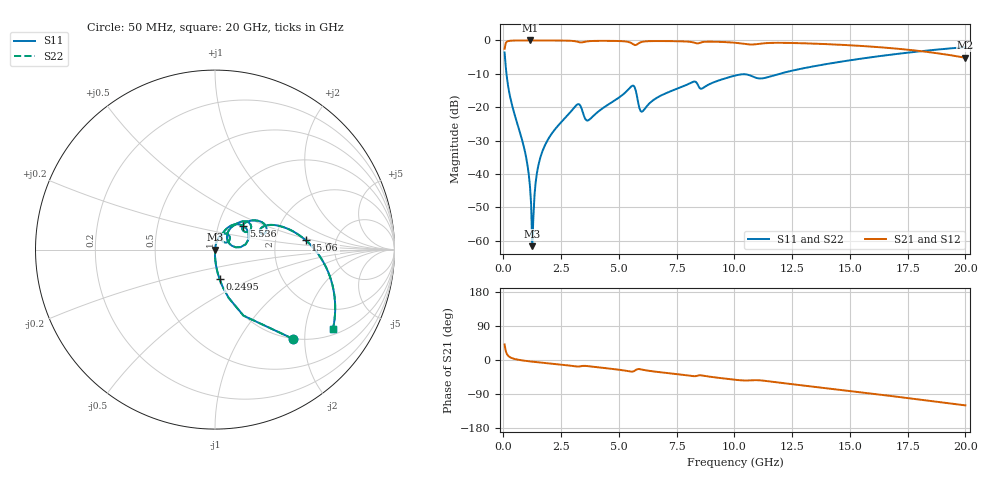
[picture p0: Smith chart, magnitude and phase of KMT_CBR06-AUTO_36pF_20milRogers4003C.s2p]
! Data measured by Modelithics Inc. support@modelithics.com 813-866-6335
! KEMET CBR06-AUTO 36pF, Pad Width= 0.851mm, Pad Length= 0.64mm, Pad Gap= 0.62mm, 20mil Rogers 4003C substrate Data, January 2022
# hz S ma R 50
! 2 Port Network Data from SP1.SP block
! freq  magS11  angS11  magS21  angS21  magS12  angS12  magS22  angS22
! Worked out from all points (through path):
!   401 points, 50 MHz to 20 GHz, reference 50 ohm
!   highest |S21| = -0.01 dB at 1.147 GHz (marker M1); lowest = -5.2 dB at 20 GHz (marker M2)
!   group delay of S21, straight-line fit = 16.7 ps
!   lowest |S11| = -61.6 dB at 1.247 GHz (marker M3), VSWR 1.00, Z = 50.1 - j0.0651 ohm
!   |S11| at or under -10 dB: 132.2 MHz to 11.95 GHz (11.82 GHz wide, 196 % of centre)
!   |S22| runs from -61.6 to -2.0 dB; largest |S21 - S12| = 0
!   S11 on the Smith chart (normalised r, x): 50 MHz: 1.00, -1.75; 249.5 MHz: 1.00, -0.34; 5.536 GHz: 1.32, +0.36; 15.06 GHz: 3.00, +0.42; 20 GHz: 1.17, -2.82
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5e7  0.6596 -48.9  0.7513 41.1  0.7513 41.1  0.6596 -48.9
2.495e8  0.167 -81.2  0.9856 8.7  0.9856 8.7  0.167 -81.2
9.4775e8  0.0203 -90.8  0.9993 -2.2  0.9993 -2.2  0.0203 -90.8
1.097375e9  0.009743 -90.3  0.9994 -3.3  0.9994 -3.3  0.009743 -90.3
1.14725e9  0.006579 -89.0  0.9994 -3.7  0.9994 -3.7  0.006579 -89.0
1.247e9  0.0008281 -51.7  0.9994 -4.4  0.9994 -4.4  0.0008281 -51.7
1.34675e9  0.004958 78.1  0.9993 -5.1  0.9993 -5.1  0.004958 78.1
1.4465e9  0.01015 80.8  0.9993 -5.7  0.9993 -5.7  0.01015 80.8
1.54625e9  0.01512 81.2  0.9992 -6.3  0.9992 -6.3  0.01512 81.2
1.8455e9  0.02912 80.2  0.9987 -8.2  0.9987 -8.2  0.02912 80.2
3.14225e9  0.1059 58.3  0.9678 -17.0  0.9678 -17.0  0.1059 58.3
3.391625e9  0.09361 32.0  0.9347 -16.0  0.9347 -16.0  0.09361 32.0
3.690875e9  0.06407 51.3  0.9738 -16.4  0.9738 -16.4  0.06407 51.3
5.53625e9  0.205 40.1  0.9134 -30.7  0.9134 -30.7  0.205 40.1
5.985125e9  0.0854 30.4  0.9489 -25.1  0.9489 -25.1  0.0854 30.4
6.73325e9  0.1441 54.1  0.9793 -31.9  0.9793 -31.9  0.1441 54.1
1.0025e10  0.2974 31.7  0.9233 -52.2  0.9233 -52.2  0.2974 31.7
1.1222e10  0.2707 22.6  0.9026 -54.3  0.9026 -54.3  0.2707 22.6
1.336662e10  0.4058 17.7  0.8977 -70.0  0.8977 -70.0  0.4058 17.7
1.506238e10  0.5078 5.9  0.8442 -82.2  0.8442 -82.2  0.5078 5.9
1.670825e10  0.608 -6.6  0.7704 -94.4  0.7704 -94.4  0.608 -6.6
2e10  0.7931 -34.1  0.5501 -119.7  0.5501 -119.7  0.7931 -34.1
